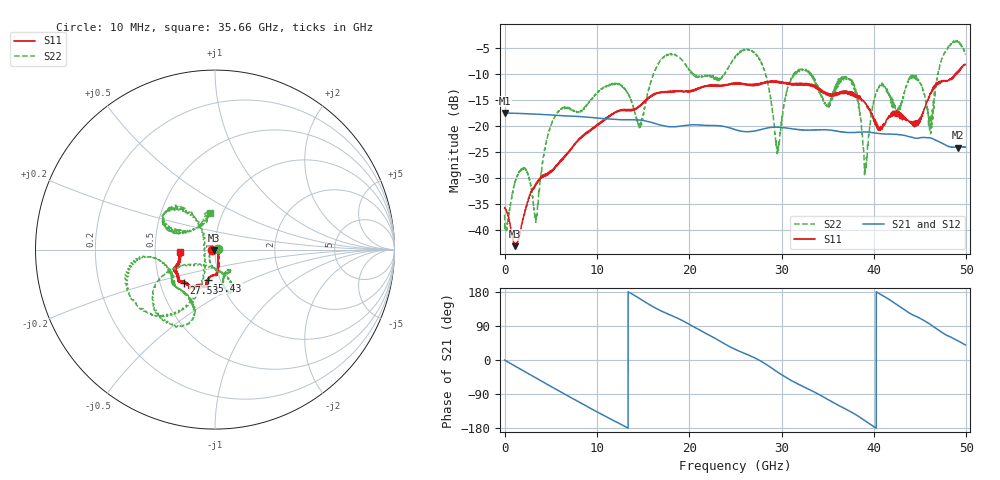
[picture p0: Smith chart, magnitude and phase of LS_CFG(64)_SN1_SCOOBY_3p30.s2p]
!Keysight Technologies,N5245B,MY58422026,A.13.80.08
!Date: Thursday, March 19, 2020 23:47:01
!Correction: S11(Full 2 Port(1,2))
!S21(Full 2 Port(1,2))
!S12(Full 2 Port(1,2))
!S22(Full 2 Port(1,2))
!S2P File: Measurements: S11, S21, S12, S22:
# Hz S DB R 50.0
!freq dBS11 angS11 dBS21 angS21 dBS12 angS12 dBS22 angS22
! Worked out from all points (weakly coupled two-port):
!   4991 points, 10 MHz to 49.91 GHz, reference 50 ohm
!   highest |S21| = -17.51 dB at 10 MHz (marker M1); lowest = -24.2 dB at 49.11 GHz (marker M2)
!   lowest |S11| = -43.0 dB at 1.12 GHz (marker M3), VSWR 1.01, Z = 49.5 - j0.466 ohm
!   |S11| at or under -10 dB: start of sweep to 48.88 GHz; 48.94765 GHz to 48.98224 GHz (34.6 MHz wide, 0.0707 % of centre)
!   |S22| runs from -40.1 to -3.6 dB; largest |S21 - S12| = 0.0012
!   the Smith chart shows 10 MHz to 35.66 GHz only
!   S11 on the Smith chart (normalised r, x): 10 MHz: 0.97, -0.01; 15.43 GHz: 0.87, -0.31; 27.53 GHz: 0.66, -0.26; 35.66 GHz: 0.68, -0.01
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1e7  -35.72 -170.2  -17.51 -0.3  -17.50 -0.3  -37.01 3.7
1.12e9  -43.03 -138.1  -17.59 -15.8  -17.58 -15.8  -30.82 -22.4
3.41e9  -31.17 -56.0  -17.75 -47.4  -17.75 -47.4  -37.99 136.5
5.26e9  -28.24 -61.4  -17.93 -73.1  -17.93 -73.0  -18.92 -88.4
8.33e9  -22.29 -75.8  -18.24 -114.5  -18.24 -114.4  -17.08 -64.6
1.543e10  -15.06 -103.7  -19.12 150.1  -19.11 150.2  -14.52 -153.7
1.665e10  -13.71 -104.1  -19.72 133.2  -19.71 133.3  -8.12 -148.0
2.496e10  -11.95 -124.5  -20.68 28.1  -20.67 28.3  -6.92 -171.1
2.753e10  -11.86 -133.2  -20.80 0.1  -20.80 0.2  -6.97 -124.1
2.956e10  -11.48 -141.1  -20.25 -31.7  -20.24 -31.6  -24.11 -178.8
3.103e10  -11.91 -145.9  -20.54 -53.8  -20.55 -53.7  -10.88 128.1
3.328e10  -12.22 -156.5  -20.79 -81.5  -20.79 -81.2  -10.52 156.6
3.566e10  -14.25 -176.9  -20.88 -112.9  -20.82 -112.5  -13.40 97.9
3.78e10  -14.20 175.5  -21.28 -140.8  -21.22 -140.9  -11.85 135.5
3.905e10  -15.50 170.6  -21.17 -160.4  -21.16 -160.6  -28.58 -126.3
4.03e10  -19.63 154.1  -21.40 179.3  -21.40 179.1  -13.35 -6.2
4.16e10  -18.17 105.0  -21.57 160.5  -21.59 160.4  -14.04 25.8
4.445e10  -19.50 53.2  -22.35 116.2  -22.37 116.5  -10.32 -15.4
4.614e10  -13.76 8.6  -22.30 93.2  -22.31 93.4  -21.06 -45.3
4.735e10  -11.33 8.4  -23.30 73.0  -23.31 73.2  -7.16 -83.2
4.911e10  -9.65 -14.2  -24.19 50.0  -24.21 50.1  -3.83 -44.3
4.991e10  -8.23 -14.9  -24.05 40.0  -24.07 40.0  -6.16 -29.0
